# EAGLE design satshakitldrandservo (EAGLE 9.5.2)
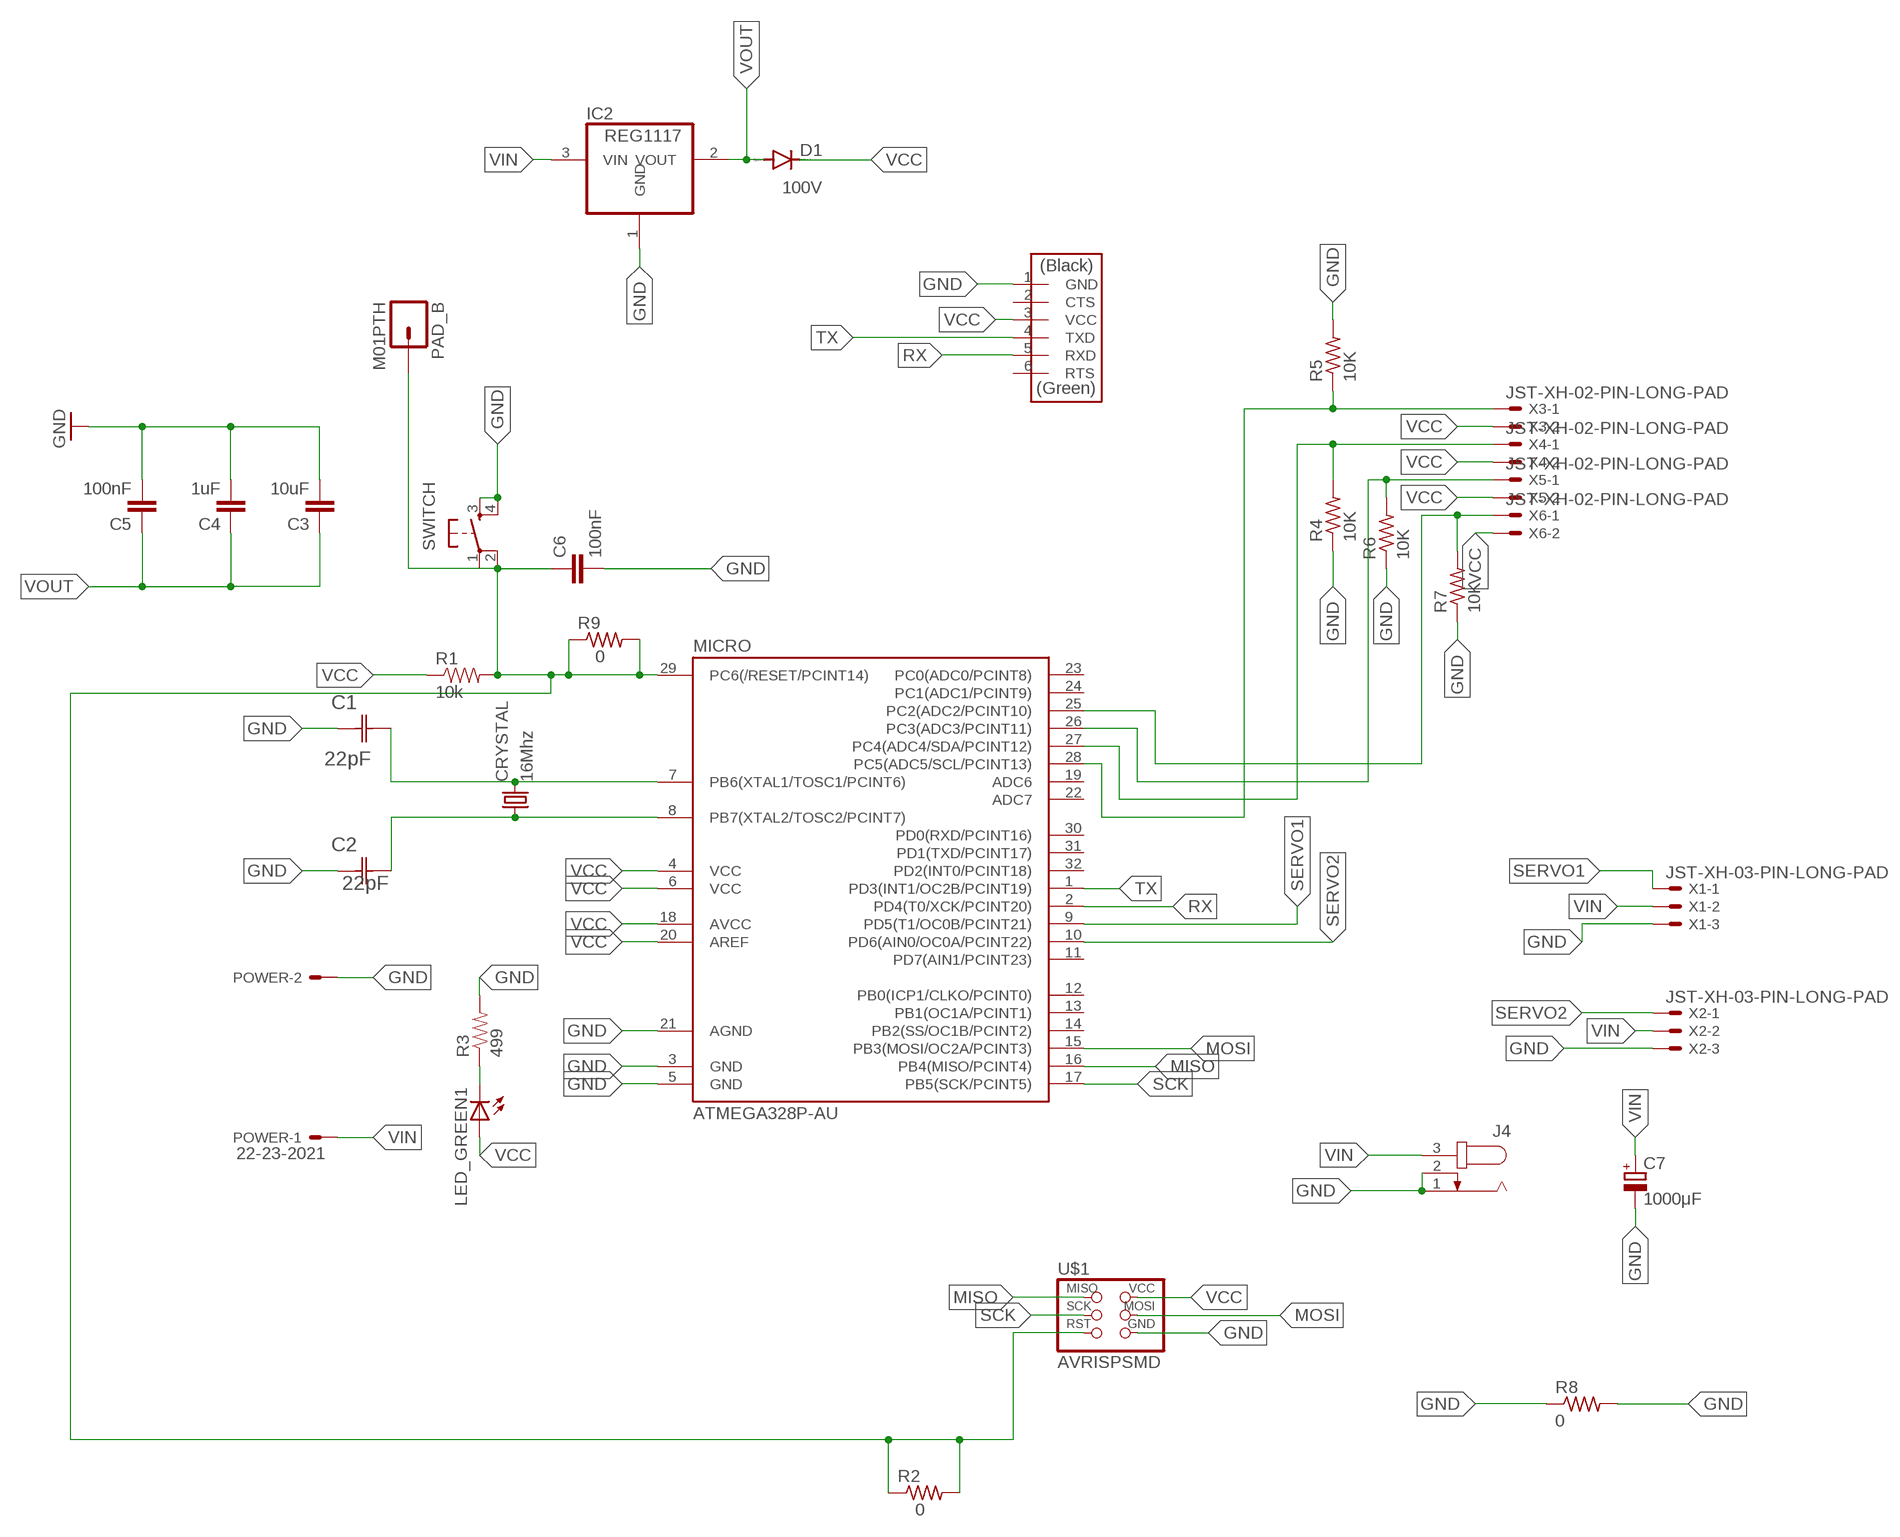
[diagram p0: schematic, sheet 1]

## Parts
C1  22pF  0612ZC225MAT2A  [CAPC3216X178N]
C2  22pF  0612ZC225MAT2A  [CAPC3216X178N]
C3  10uF  CAP1206  [1206]
C4  1uF  CAP1206  [1206]
C5  100nF  CAP1206  [1206]
C6  100nF  CAP1206  [1206]
C7  1000μF  CPOL-EUE5-10.5  [E5-10,5]
CRYSTAL  16Mhz  CSM-7X-DU  [CSM-7X-DU]
D1  100V  1N4004  [DO41-10]
IC2  REG1117  [SOT223]
J4  JACK-PLUG1  [SPC4078]
LED_GREEN1  LED1206  [1206]
MICRO  ATMEGA328P-AU  ATMEGA48/88/168-AU  [TQFP32-08]
PAD_B  M01PTH  [1X01]
POWER  22-23-2021  [22-23-2021]
R1  10k  RESISTOR1206  [1206]
R2  0  RES-US1206  [R1206]
R3  499  RESISTOR1206  [1206]
R4  10K  RES-US1206  [R1206]
R5  10K  RES-US1206  [R1206]
R6  10K  RES-US1206  [R1206]
R7  10K  RES-US1206  [R1206]
R8  0  RES-US1206  [R1206]
R9  0  RES-US1206  [R1206]
SWITCH  6MM_SWITCH6MM_SWITCH  [6MM_SWITCH]
U$1  AVRISPSMD  [2X03SMD]
U$2  FTDI-SMD-HEADER  [1X06SMD]
X1  JST-XH-03-PIN-LONG-PAD  [JST-XH-03-PACKAGE-LONG-PAD]
X2  JST-XH-03-PIN-LONG-PAD  [JST-XH-03-PACKAGE-LONG-PAD]
X3  JST-XH-02-PIN-LONG-PAD  [JST-XH-02-PACKAGE-LONG-PAD]
X4  JST-XH-02-PIN-LONG-PAD  [JST-XH-02-PACKAGE-LONG-PAD]
X5  JST-XH-02-PIN-LONG-PAD  [JST-XH-02-PACKAGE-LONG-PAD]
X6  JST-XH-02-PIN-LONG-PAD  [JST-XH-02-PACKAGE-LONG-PAD]

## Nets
GND: C1.1(C1) C2.1(C1) C3.2 C4.2 C5.2 C6.2 C7.- IC2.1(GND) J4.1 J4.2 MICRO.3(GND) MICRO.5(GND) MICRO.21(AGND) POWER.2 R3.2 R4.1 R5.2 R6.1 R7.1 R8.1 R8.2 SWITCH.3(S) SWITCH.4(S1) U$1.6(GND) U$2.1(GND) X1.3 X2.3
MISO: MICRO.16(PB4(MISO/PCINT4)) U$1.1(MISO)
MOSI: MICRO.15(PB3(MOSI/OC2A/PCINT3)) U$1.4(MOSI)
N$1: LED_GREEN1.2(C) R3.1
N$2: C1.2(C2) CRYSTAL.2 MICRO.7(PB6(XTAL1/TOSC1/PCINT6))
N$9: C2.2(C2) CRYSTAL.1 MICRO.8(PB7(XTAL2/TOSC2/PCINT7))
N$17: C6.1 MICRO.29(PC6(/RESET/PCINT14)) PAD_B.1 R1.2 R2.1 R2.2 R9.1 R9.2 SWITCH.1(P) SWITCH.2(P1) U$1.5(RST)
N$18: MICRO.27(PC4(ADC4/SDA/PCINT12)) R4.2 X4.1
N$20: MICRO.26(PC3(ADC3/PCINT11)) R6.2 X5.1
N$25: MICRO.25(PC2(ADC2/PCINT10)) R7.2 X6.1
N$29: MICRO.28(PC5(ADC5/SCL/PCINT13)) R5.1 X3.1
RX: MICRO.2(PD4(T0/XCK/PCINT20)) U$2.5(RXD)
SCK: MICRO.17(PB5(SCK/PCINT5)) U$1.3(SCK)
SERVO1: MICRO.9(PD5(T1/OC0B/PCINT21)) X1.1
SERVO2: MICRO.10(PD6(AIN0/OC0A/PCINT22)) X2.1
TX: MICRO.1(PD3(INT1/OC2B/PCINT19)) U$2.4(TXD)
VCC: D1.C LED_GREEN1.1(A) MICRO.4(VCC) MICRO.6(VCC) MICRO.18(AVCC) MICRO.20(AREF) R1.1 U$1.2(VCC) U$2.3(VCC) X3.2 X4.2 X5.2 X6.2
VIN: C7.+ IC2.3(VIN) J4.3 POWER.1 X1.2 X2.2
VOUT: C3.1 C4.1 C5.1 D1.A IC2.2(VOUT)
Unconnected: MICRO.11(PD7(AIN1/PCINT23)) MICRO.12(PB0(ICP1/CLKO/PCINT0)) MICRO.13(PB1(OC1A/PCINT1)) MICRO.14(PB2(SS/OC1B/PCINT2)) MICRO.19(ADC6) MICRO.22(ADC7) MICRO.23(PC0(ADC0/PCINT8)) MICRO.24(PC1(ADC1/PCINT9)) MICRO.30(PD0(RXD/PCINT16)) MICRO.31(PD1(TXD/PCINT17)) MICRO.32(PD2(INT0/PCINT18)) U$2.2(CTS) U$2.6(RTS)

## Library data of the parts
C1 C2 = AVX_By_element14_Batch_1:0612ZC225MAT2A: Capacitor 1206; MPN: 0612ZC225MAT2A; OC_FARNELL: -; OC_NEWARK: 12N3209; SUPPLIER: AVX; TOLERANCE: ±20%; VALUE: 2.2µF; VOLTAGERATING: 10V
C3-C6 = 01_SparkFun:CAP: Capacitor
C7 = rcl:CPOL-EU: POLARIZED CAPACITOR, European symbol; SPICEPREFIX: C
CRYSTAL = 01_FAB_Hello:CSM-7X-DU: SMD CRYSTAL; OC_FARNELL: unknown; OC_NEWARK: unknown
D1 = diode:1N4004: DIODE
IC2 = burr-brown:REG1117: 800mA and 1A Low Dropout (LDO) Positive Regulator 1.8V, 2.5V, 2.85V, 3.3V, 5V, and Adj; MPN: REG1117; OC_FARNELL: 1097566; OC_NEWARK: 14P6981
J4 = con-jack:JACK-PLUG: DC POWER JACK Power Jack, DC, Right Angle, Through Hole, Rated 5A at 16VDC, PC Terminals Distributor: Farnell (www.Farnell.de) Drawing: 84N1161.pdf / 84N1162.pdf Manufacturer: SPC Technology (www.spctechnology.com) Type: SPC4077 / SPC 4078; OC_FARNELL: unknown; OC_NEWARK: unknown
LED_GREEN1 = 01_FAB_Hello:LED
MICRO = atmega8:ATMEGA48/88/168
PAD_B = 01_SparkFun:M01: Header 1
POWER = con-molex:22-23-2021: .100" (2.54mm) Center Header - 2 Pin; MF: MOLEX; MPN: 22-23-2021; OC_FARNELL: 1462926; OC_NEWARK: 25C3832
R1 R3 = 01_SparkFun:RESISTOR: Resistor
R2 R4-R9 = files_fab:RES-US: Resistor (US Symbol)
SWITCH = 01_FAB_Hello:6MM_SWITCH: OMRON SWITCH
U$1 = files_fab:AVRISP
U$2 = fab:FTDI-SMD-HEADER
X1 X2 = Rembrandt Electronics - JST XH Connectors v1-0 (1):JST-XH-03-PIN: JST XH Connector 2 Pin Wire to board connector. Pitch: 2,54 mm, (0.100") Number of pins: 3 Created by Rembrandt Electronics www.rembrandtelectronics.com
X3-X6 = Rembrandt Electronics - JST XH Connectors v1-0 (1):JST-XH-02-PIN: JST XH Connector 2 Pin

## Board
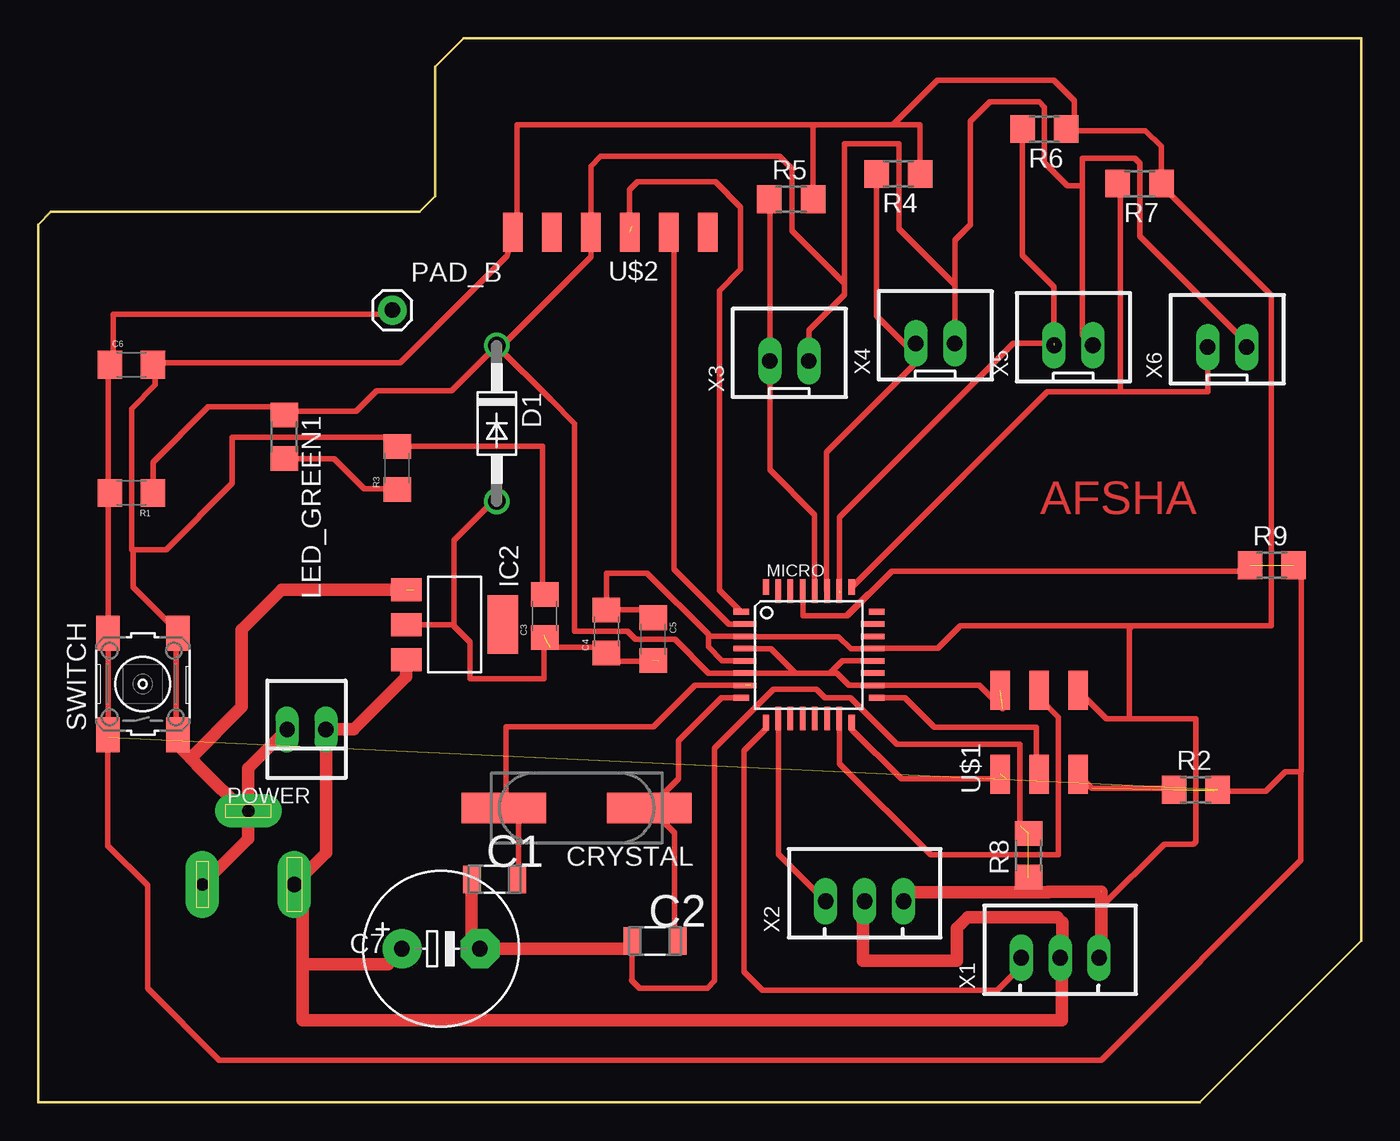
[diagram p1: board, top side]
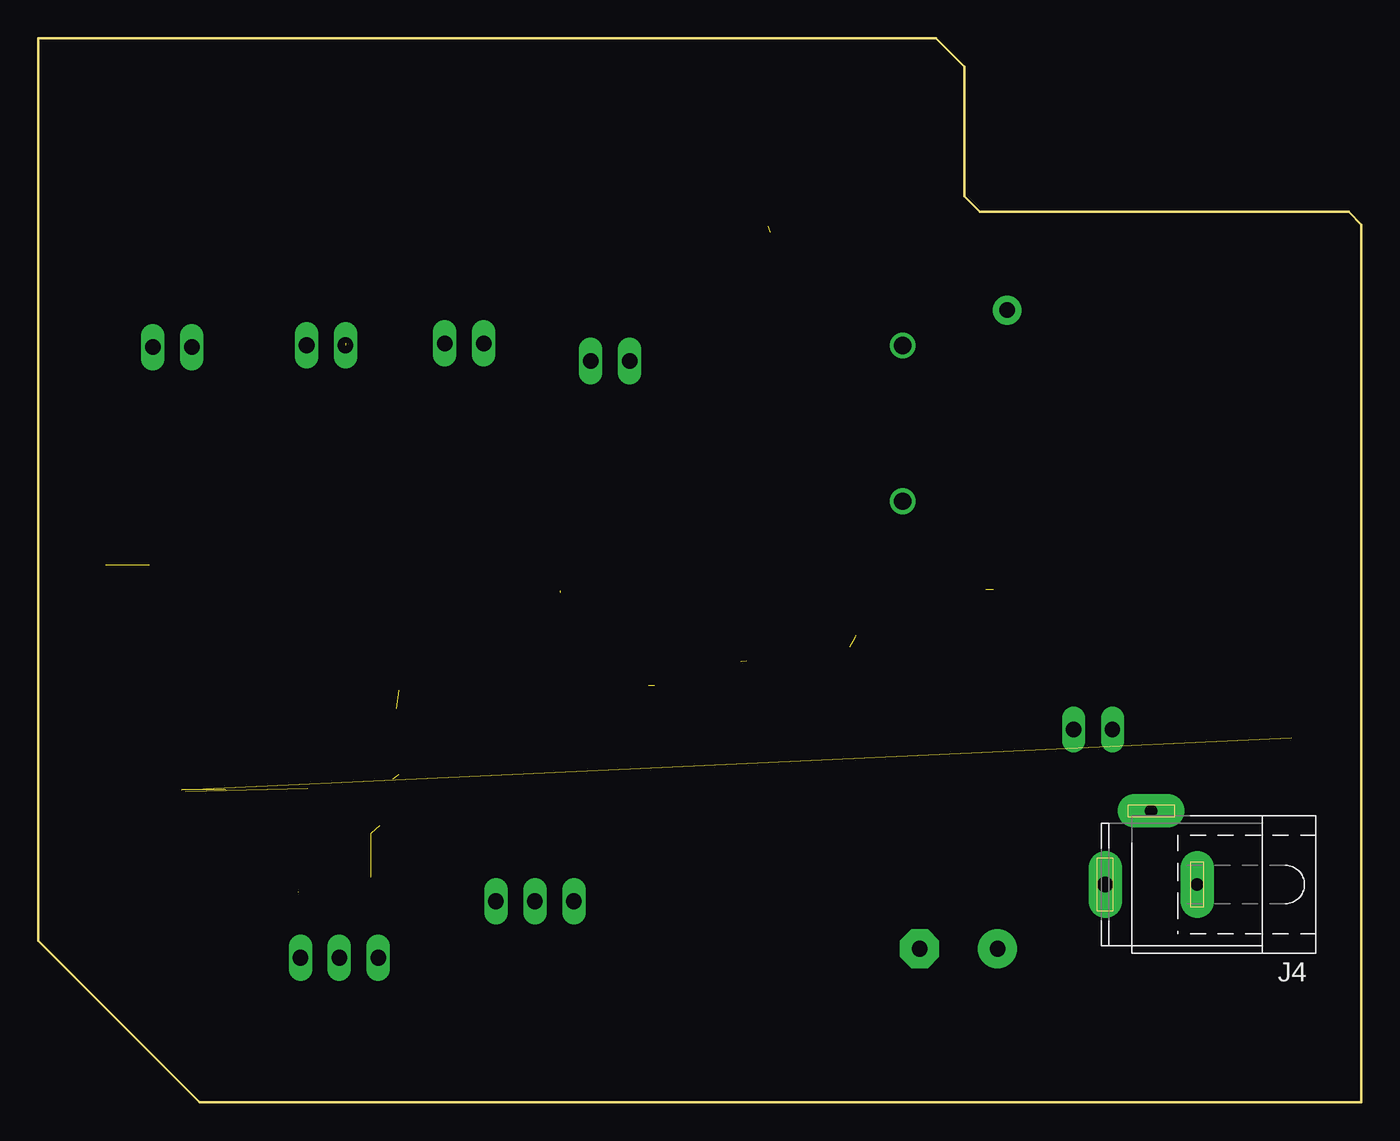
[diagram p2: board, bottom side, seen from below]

Size 86.33 x 69.41 mm. Coordinates in mm from the lower left corner, seen from the top.
Outline: 0,0.02 0,57.26 0.82,58.08 24.87,58.08 25.9,59.11 25.9,67.55 27.75,69.41 86.33,69.41 86.33,10.53 75.8,0 0,0
Copper layers (1*16): Top 0.035mm / dielectric 1.5mm / Bottom 0.035mm
Design rules "default *": minimum track width 14mil, minimum drill 24mil, track to track 16mil, track to pad 16mil, pad to pad 16mil, via to via 16mil, smd to smd 16mil, copper to edge 40mil, drill to drill 14mil, minimum pad ring 10mil, minimum via ring 8mil, stop-mask expansion 4mil, vias tented up to drill 0mil, thermal gap 10mil

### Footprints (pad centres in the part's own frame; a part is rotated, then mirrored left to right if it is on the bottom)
CAPC3216X178N = smd 1.118 x 1.803: 1 -1.499,0; 2 1.499,0
1206 = smd 1.6 x 1.8: 1 -1.4,0; 2 1.4,0
E5-10,5 = drill 1.016 pad 2.54: + -2.54,0 | drill 1.016 pad 2.54 octagon: - 2.54,0
CSM-7X-DU = smd 5.5 x 2: 1 -4.75,0; 2 4.75,0
DO41-10 = drill 1.118: A 5.08,0; C -5.08,0
SOT223 = smd 1.499 x 2.007: 1 -2.261,-3.15; 2 0.025,-3.15; 3 2.311,-3.15 | smd 3.81 x 2.007: 4 0,3.15
SPC4078 = drill 0.8 pad 2.184 long: 1 -3,0; 2 0,-4.8 | drill 1 pad 2.184 long: 3 3,0
1206' = smd 1.6 x 1.803: 1 -1.422,0; 2 1.422,0
TQFP32-08 = smd 1.016 x 0.406: 1 -4.42,2.8; 8 -4.42,-2.8; 17 4.42,-2.8; 24 4.42,2.8 | smd 1.524 x 0.356: 2 -4.166,2; 3 -4.166,1.2; 4 -4.166,0.4; 5 -4.166,-0.4; 6 -4.166,-1.2; 7 -4.166,-2; 18 4.166,-2; 19 4.166,-1.2; 20 4.166,-0.4; 21 4.166,0.4; 22 4.166,1.2; 23 4.166,2 | smd 0.406 x 1.016: 9 -2.8,-4.42; 16 2.8,-4.42; 25 2.8,4.42; 32 -2.8,4.42 | smd 0.356 x 1.524: 10 -2,-4.166; 11 -1.2,-4.166; 12 -0.4,-4.166; 13 0.4,-4.166; 14 1.2,-4.166; 15 2,-4.166; 26 2,4.166; 27 1.2,4.166; 28 0.4,4.166; 29 -0.4,4.166; 30 -1.2,4.166; 31 -2,4.166
1X01 = drill 1.016 pad 1.88: 1 0,0
22-23-2021 = drill 1 long: 1 -1.27,0; 2 1.27,0
R1206 = smd 1.6 x 1.803: 1 -1.422,0; 2 1.422,0
6MM_SWITCH = smd 2.286 x 1.524: 1 -3.302,2.286; 2 3.302,2.286; 3 -3.302,-2.286; 4 3.302,-2.286
2X03SMD = smd 2.54 x 1.27: 1 -2.54,2.54; 2 2.92,2.54; 3 -2.54,0; 4 2.92,0; 5 -2.54,-2.54; 6 2.92,-2.54
1X06SMD = smd 2.54 x 1.27: 1 0,6.35; 2 0,3.81; 3 0,1.27; 4 0,-1.27; 5 0,-3.81; 6 0,-6.35
JST-XH-03-PACKAGE-LONG-PAD = drill 1.016 long: 1 -2.54,0; 2 0,0; 3 2.54,0
JST-XH-02-PACKAGE-LONG-PAD = drill 1.016 long: 1 -1.27,0; 2 1.27,0

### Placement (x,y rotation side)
C1  29.77,14.54 0 top
C2  40.25,10.51 0 top
C3  33.04,31.71 90 top
C4  37.07,30.71 90 top
C5  40.12,30.21 90 top
C6  6.08,48.11 0 top
C7  26.28,10.01 0 top
CRYSTAL  35.13,19.2 180 top
D1  29.92,44.28 270 top
IC2  27.16,31.17 270 top
J4  13.7,14.2 180 bottom
LED_GREEN1  [1206']  16.05,43.4 270 top
MICRO  50.28,29.19 0 top
PAD_B  23.1,51.67 0 top
POWER  17.5,24.32 180 top
R1  6.08,39.76 180 top
R2  75.54,20.39 0 top
R3  23.43,41.38 90 top
R4  56.12,60.56 180 top
R5  49.14,58.91 0 top
R6  65.65,63.48 180 top
R7  71.87,59.92 180 top
R8  64.62,16.11 90 top
R9  80.51,35.03 0 top
SWITCH  6.82,27.28 90 top
U$1  65.31,23.95 90 top
U$2  37.33,56.75 90 top
X1  66.68,9.43 0 top
X2  53.92,13.11 0 top
X3  49.01,48.37 0 top
X4  58.53,49.51 0 top
X5  67.55,49.38 0 top
X6  77.58,49.26 0 top

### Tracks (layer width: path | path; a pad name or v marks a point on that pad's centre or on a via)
GND  (5 unrouted)
  Top 0.356: 38.25,10.01 C2.1 38.75,7.98 38.73,7.97 39.25,7.45 43.67,7.45 44.14,7.92 44.14,23.08 47.99,26.93 50.79,26.93 51.33,26.39 53,26.39 56.02,23.36 64.06,23.36 64.06,18.04 | 40.06,31.67 C5.2 39.61,32.11 C4.2 37.07,34.52 39.73,34.52 43.73,30.52 | R5.2 50.79,59.03 50.56,59.26 50.56,63.63 50.69,63.76 | 57.26,60.3 R4.1 57.52,60.58 57.52,63.76 55.77,63.76 | 6.2,36.05 6.2,33.58 9,30.78 SWITCH.4 9,30.46 9,24.11 SWITCH.3 | 54.99,29.6 58.69,29.6 60.18,31.09 71.4,31.09 | 54.99,29.6 54.46,29.6 MICRO.21 | 71.4,31.09 80.48,31.09 80.48,52.65 73.46,59.67 R7.1 73.29,62.35 72.26,63.39 67.16,63.39 R6.1 67.38,63.48 67.62,63.72 67.62,65.34 66.28,66.67 58.68,66.67 55.77,63.76 | 50.69,63.76 55.77,63.76 | C1.1 28.42,14.68 | 28.69,10.01 C7.- 28.28,10.55 | 50.69,63.76 31.23,63.76 31.23,56.81 U$2.1 30.6,55.23 23.61,48.24 7.73,48.24 C6.2 7.63,47.96 7.63,46.8 6.08,45.25 6.08,36.05 6.2,36.05 | MICRO.5 46.1,28.79 46.08,28.81 44.63,28.81 43.73,29.71 43.73,30.52 | 54.99,29.6 54.97,29.59 53.02,29.59 52.23,30.38 46.15,30.38 46.14,30.39 MICRO.3 46.1,30.41 43.84,30.41 43.73,30.52 | 69.38,9.59 X1.3 | C3.2 32.89,33.26 32.89,42.8 27.6,42.8 27.65,42.78 R3.2 23.34,42.6 22.55,43.39 12.65,43.39 12.65,40.37 8.33,36.05 6.2,36.05 | 71.2,25.01 75.54,25.01 75.54,21.51 75.54,16.99 75.38,16.83 73.47,16.83 69.38,12.75 | 71.2,25.01 69.71,25.01 U$1.6 | 71.2,25.01 71.2,30.89 71.4,31.09 | 65.9,13.69 65.87,13.72 | 64.78,14.82 64.61,14.98 | R8.1 64.62,13.84 64.47,13.69
  Top 0.406: X2.3 56.62,13.27
  Top 0.813: C7.- 38.25,10.01 | 9.94,22.44 10.64,21.74 13.38,19 J4.2 | 9.94,22.44 9.11,23.28 SWITCH.3 | J4.1 13.7,17.2 J4.2 | X2.3 57.04,13.69 64.47,13.69 65.9,13.69 | 65.87,13.72 69.34,13.72 | 69.38,13.72 69.38,12.75 69.38,9.59 | J4.2 13.7,21.79 POWER.2 | C1.1 28.28,10.55 | 9.94,22.44 13.28,25.79 13.28,30.83 15.87,33.42 24.48,33.42
MISO  (1 unrouted)
  Top 0.356: MICRO.16 53.08,24.33 56.32,21.09 63.17,21.09
MOSI
  Top 0.356: MICRO.15 52.29,25.01 52.29,22.09 58.24,16.14 66.58,16.14 66.58,25.12 65.31,26.38 U$1.4
N$1
  Top 0.356: R3.1 23.4,40.02 21.27,40.02 19.31,41.98 LED_GREEN1.2
N$2  (1 unrouted)
  Top 0.356: C1.2 31.34,14.48 31.34,18.24 CRYSTAL.2 30.52,19.34 30.52,24.49 40.14,24.49 42.85,27.2 46.5,27.2
N$3
  Bottom 0.356: 10.68,15.4 10.68,13.07
N$4
  Bottom 0.356: 16.66,15.7 16.66,12.82
N$5
  Bottom 0.356: 12.46,19.03 14.85,19.03
N$9
  Top 0.356: MICRO.8 44.59,26.39 41.79,23.59 41.79,21.11 CRYSTAL.1 41.51,17.57 41.51,10.75 C2.2
N$17  (4 unrouted)
  Top 0.356: PAD_B.1 22.97,51.41 4.88,51.41 4.88,48.24 C6.1 4.56,47.92 4.56,39.98 R1.2 4.56,39.67 4.56,30.78 SWITCH.2 4.56,30.46 4.56,24.11 SWITCH.1 | 4.56,23.79 SWITCH.1 | 52.74,31.73 52.79,31.73 55.71,34.65 78.7,34.65 R9.1 | R9.2 82.18,34.78 82.41,34.78 82.41,21.58 82.4,21.58 82.4,21.55 | SWITCH.1 4.53,16.74 7.12,14.15 7.12,7.43 11.81,2.74 69.37,2.74 82.4,15.77 82.4,21.55 | 49.89,31.73 49.89,33.34 MICRO.29 49.89,33.35 49.89,31.73 | 49.89,31.73 52.74,31.73 | 52.74,31.73 54.16,33.16 | 82.4,21.55 81.37,21.55 80.1,20.28 76.7,20.28 | 74.4,20.49 68.77,20.49 U$1.5
N$18
  Top 0.356: MICRO.27 51.44,33.39 51.44,42.42 57.52,48.49 56.88,49.13 | X4.1 56.88,49.13 | R4.2 54.7,51.31 56.88,49.13
N$20  (2 unrouted)
  Top 0.356: R6.2 64.22,55.25 66.28,53.19 X5.1 | 52.28,33.25 52.28,38.17 63.62,49.51 66.29,49.51
N$25
  Top 0.356: 70.6,46.33 76.31,46.33 X6.1 | 70.6,46.33 65.84,46.33 53.14,33.63 MICRO.25 | 70.6,46.33 70.6,59.67 R7.2
N$29
  Top 0.356: MICRO.28 50.66,33.38 50.66,38.34 47.74,41.25 X3.1 47.74,58.89 R5.1
RX
  Top 0.356: U$2.5 41.5,56.39 41.5,34.76 45.07,31.19 MICRO.2
SCK
  Top 0.356: MICRO.17 56.55,26.39 58.48,24.46 65.15,24.46 65.15,21.57 U$1.3
SERVO1
  Top 0.356: X1.1 64.14,8.86 62.58,7.3 47.25,7.3 46.05,8.5 46.05,22.94 47.48,24.36 MICRO.9
SERVO2
  Top 0.356: X2.1 48.31,16.19 48.31,24.99 MICRO.10
TX  (1 unrouted)
  Top 0.356: 38.72,57.13 38.72,57.26 38.6,57.13 38.6,59.54 39.1,60.05 44.18,60.05 45.83,58.4 45.83,54.34 44.44,52.94 44.44,33.41 MICRO.1
VCC  (1 unrouted)
  Top 0.356: 68.12,59.8 68.12,50.08 X5.2 | 68.12,59.8 68.12,61.57 71.55,61.57 71.87,61.26 71.87,56.49 78.85,49.51 X6.2 | 51.66,27.97 52.13,27.97 52.91,27.19 MICRO.18 61.41,27.19 62.94,25.67 | 49.42,27.97 48.96,27.97 48.94,27.99 MICRO.6 43.75,27.99 41.54,30.2 38.98,30.2 38.47,30.72 35.01,30.72 35.01,44.28 33.46,45.82 | 51.66,27.97 49.42,27.97 | MICRO.20 52.48,28.79 51.66,27.97 | D1.C 30.26,49.36 36.06,55.16 U$2.3 36.06,61.07 36.69,61.7 48.37,61.7 49.17,60.9 49.17,56.84 52.6,53.41 | R1.1 7.48,41.77 11.1,45.38 16.67,45.38 LED_GREEN1.1 16.12,45.06 20.75,45.06 22.09,46.4 26.96,46.4 D1.C | 33.46,45.82 | D1.C 33.46,45.82 | 59.8,53.32 59.8,56.24 60.82,57.26 60.82,63.98 62.09,65.25 65.32,65.25 65.67,64.9 65.67,61.3 67.17,59.8 68.12,59.8 | 59.8,53.32 X4.2 | 59.8,53.32 56.16,56.97 56.16,62.52 52.6,62.52 52.6,53.41 | 52.6,53.41 52.6,52.67 50.28,50.35 X3.2 | MICRO.4 47.81,29.59 49.42,27.97
VIN
  Top 0.356: 17.39,9 17.26,9.12 | 66.81,9.3 X1.2 | 53.82,13.01 X2.2
  Top 0.813: C7.+ 23.74,9.91 22.83,9 17.39,9 | 66.81,9.3 66.81,5.36 17.26,5.36 17.26,9.12 17.26,13.65 J4.3 18.77,16.27 POWER.1 20.59,24.32 24.01,27.75 IC2.3 | X1.2 66.83,9.57 66.83,11.75 66.51,12.06 60.67,12.06 59.96,11.35 59.96,9.22 53.82,9.22 53.82,13.01
VOUT  (3 unrouted)
  Top 0.356: 29.92,38.82 D1.A 29.69,39.2 27.13,36.65 27.13,31.14 27.05,31.14 | 33.39,29.69 36.69,29.69 C4.1 37.6,28.78 40.48,28.78 | 27.05,31.14 IC2.2 | 27.05,31.14 28.18,30.01 28.18,27.64 33.01,27.64 33.01,30.45

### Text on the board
Top: AFSHA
